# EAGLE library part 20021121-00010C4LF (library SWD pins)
Headers & Wire Housings 1.27x1.27mm BTB, Hdr Unshrd, SMT, 10 Pos Source: Datasheet
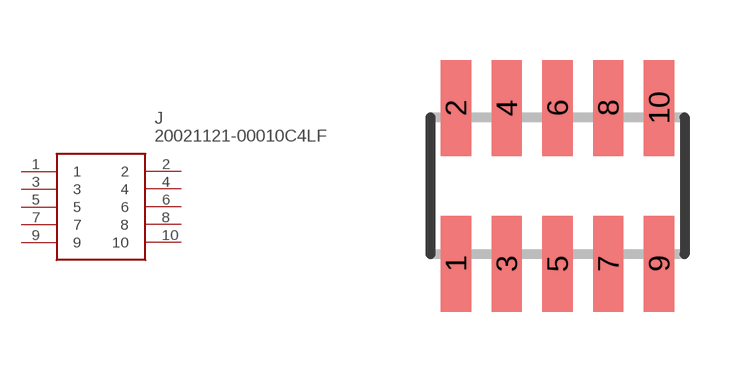
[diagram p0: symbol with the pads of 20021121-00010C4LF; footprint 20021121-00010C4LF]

Designator prefix J

## 20021121-00010C4LF (ALLIED_NUMBER: 70247660; ALLIED_PRICE-STOCK: http://www.alliedelec.com/fci-20021121-00010c4lf/70247660/; DESCRIPTION: Headers & Wire Housings 1.27x1.27mm BTB, Hdr Unshrd, SMT, 10 Pos; HEIGHT: mm; MANUFACTURER_NAME: FCI; MANUFACTURER_PART_NUMBER: 20021121-00010C4LF; MOUSER_PART_NUMBER: 649-202112100010C4LF; MOUSER_PRICE-STOCK: https://www.mouser.com/Search/Refine.aspx?Keyword=649-202112100010C4LF; RS_PART_NUMBER: 1708866; RS_PRICE-STOCK: http://uk.rs-online.com/web/p/products/1708866)  [20021121-00010C4LF]
1  1
2  2
3  3
4  4
5  5
6  6
7  7
8  8
9  9
10  10

## Footprint 20021121-00010C4LF (pad centres in mm)
20021121-00010C4LF
smd 0.76 x 2.4: 1 -2.54,-1.95; 2 -2.54,1.95; 3 -1.27,-1.95; 4 -1.27,1.95; 5 0,-1.95; 6 0,1.95; 7 1.27,-1.95; 8 1.27,1.95; 9 2.54,-1.95; 10 2.54,1.95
